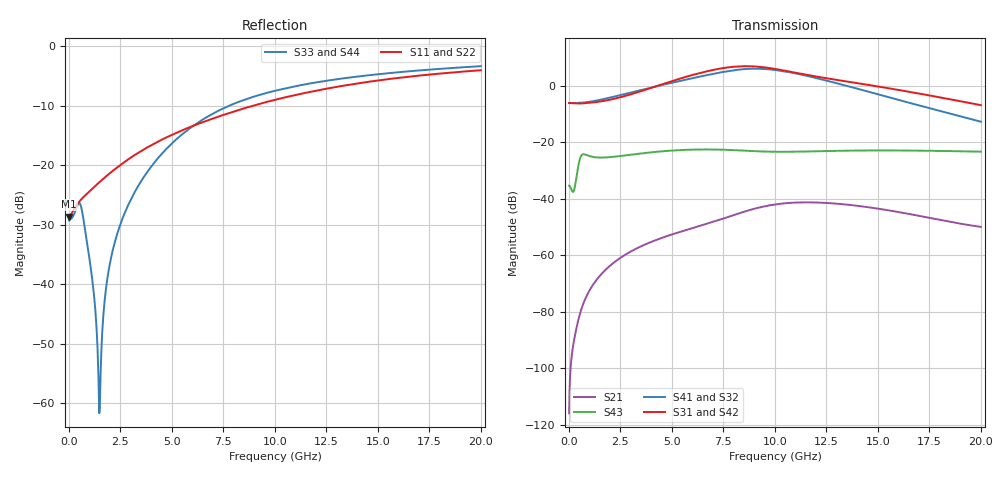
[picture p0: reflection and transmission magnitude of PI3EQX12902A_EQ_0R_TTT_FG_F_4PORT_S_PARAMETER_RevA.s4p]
! NPort=4 DATA=2000 NOISE=0 GROUPDELAY=0 COMPLEX_DATAFORMAT=POLAR
! NumOfBlock=1 NumOfParam=0
! .MODEL Smodel S TSTONEFILE=PI3EQX12902A_EQ_0R_TTT_FG_F_4PORT_S_PARAMETER_RevA.s4p TYPE=S
!  -- The above .MODEL line can be used for the S element in the netlist.
! The s parameter is extracted from the linear redriver, it is not bi-directional; only s(4,1)s(4,2) and s(3,1)s(3,2)
! should be the insertion loss
!Port definition:
!Port1 = input+
!Port2 = input-
!Port3 = output+
!Port4 = output-
# Hz S MA R  50
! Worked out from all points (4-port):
!   2000 points, 10 MHz to 20 GHz, reference 50 ohm
!   strongest paths, dB at 10 MHz, 5.01 GHz, 10.01 GHz, 15.01 GHz, 20 GHz:
!     S31: -6.0, 1.7, 6.0, -0.2, -6.8
!     S42: -6.0, 1.6, 5.8, -0.4, -7.0
!     S41: -6.0, 1.1, 5.7, -3.0, -12.7
!     S32: -6.0, 1.2, 5.6, -3.1, -12.8
!     S43: -35.3, -22.9, -23.3, -22.9, -23.3
!     S21: -116.0, -52.6, -42.0, -43.5, -49.9
!   lowest |S11| = -28.6 dB at 10 MHz (marker M1), VSWR 1.08, Z = 46.4 - j0.0607 ohm
!   |S11| at or under -10 dB: start of sweep to 8.936 GHz
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1e7  0.03704 -179.0  1.583e-06 51.7  0 0.0  0 0.0
     1.583e-06 51.7  0.03704 -179.0  0 0.0  0 0.0
     0.4985 -0.1  0.4985 179.9  0.03429 6.0  0.01709 -177.1
     0.4985 179.9  0.4985 -0.1  0.01709 -177.1  0.03429 6.0
1.49e9  0.0722 -133.4  0.0004275 115.2  3.743e-09 177.1  5.622e-09 -173.9
        0.0004275 115.2  0.0722 -133.4  5.623e-09 -173.8  3.745e-09 177.2
        0.5283 2.9  0.567 176.8  0.0008858 -60.3  0.05389 -174.9
        0.5652 176.7  0.5283 2.6  0.05389 -174.8  0.0009453 -62.8
6.1e9  0.2167 -112.3  0.003098 77.7  1.785e-06 -25.5  1.092e-06 84.7
       0.003101 77.7  0.2167 -112.3  1.099e-06 84.9  1.78e-06 -25.4
       1.601 -40.6  1.397 105.3  0.2182 -47.6  0.07414 143.5
       1.396 105.5  1.573 -41.2  0.07454 143.6  0.2176 -47.6
8.24e9  0.2908 -112.3  0.005479 60.0  7.493e-06 -88.1  4.741e-06 30.1
        0.0055 60.0  0.2909 -112.3  4.795e-06 30.1  7.484e-06 -88.0
        2.221 -96.2  1.943 47.1  0.3404 -68.1  0.07178 121.9
        1.944 47.2  2.179 -96.6  0.07223 121.8  0.3398 -68.0
1.161e10  0.4099 -116.5  0.008611 2.1  2.061e-05 -174.4  1.479e-05 -79.9
          0.008657 1.8  0.4099 -116.5  1.495e-05 -80.4  2.057e-05 -174.4
          1.558 179.8  1.485 -60.0  0.4827 -90.7  0.06893 101.6
          1.491 -59.7  1.52 179.4  0.06907 101.3  0.4829 -90.6
1.453e10  0.5018 -121.8  0.007083 -39.1  3.3e-05 131.3  1.86e-05 -153.4
          0.007096 -39.9  0.5017 -121.8  1.877e-05 -154.0  3.289e-05 131.4
          1.044 130.2  0.7844 -128.7  0.5694 -103.8  0.07182 81.6
          0.7928 -128.5  1.016 130.3  0.0718 81.4  0.57 -103.8
2e10  0.6281 -131.4  0.00328 -65.6  4.634e-05 49.3  1.722e-05 112.3
      0.003181 -66.4  0.6281 -131.4  1.736e-05 111.3  4.617e-05 49.6
      0.4565 50.3  0.2282 140.0  0.6795 -119.6  0.0685 46.2
      0.2325 139.7  0.4464 50.7  0.06846 46.2  0.6798 -119.6
